FUNCTION "Gest Output" : VOID
TITLE =GESTIONE OUTPUT
AUTHOR : MassimoZ
VERSION : 0.1

BEGIN
NETWORK
TITLE =Spia Manuale
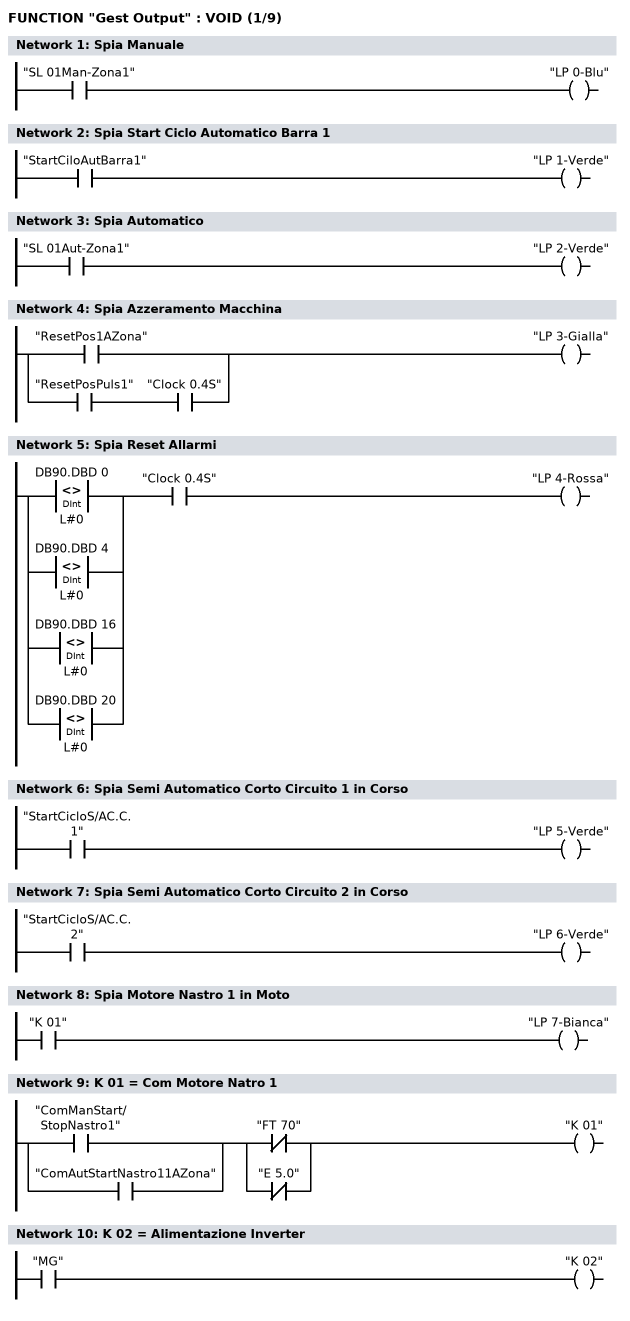
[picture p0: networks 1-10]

      U     "SL 01Man-Zona1";
      =     "LP 0-Blu";
NETWORK
TITLE =Spia Start Ciclo Automatico Barra 1

      U     "StartCiloAutBarra1";
      =     "LP 1-Verde";
NETWORK
TITLE =Spia Automatico

      U     "SL 01Aut-Zona1";
      =     "LP 2-Verde";
NETWORK
TITLE =Spia Azzeramento Macchina

      O     "ResetPos1AZona";
      O     ;
      U     "ResetPosPuls1";
      U     "Clock 0.4S";
      =     "LP 3-Gialla";
NETWORK
TITLE =Spia Reset Allarmi

      U(    ;
      O(    ;
      L     DB90.DBD    0;
      L     L#0;
      <>D   ;
      )     ;
      O(    ;
      L     DB90.DBD    4;
      L     L#0;
      <>D   ;
      )     ;
      O(    ;
      L     DB90.DBD   16;
      L     L#0;
      <>D   ;
      )     ;
      O(    ;
      L     DB90.DBD   20;
      L     L#0;
      <>D   ;
      )     ;
      )     ;
      U     "Clock 0.4S";
      =     "LP 4-Rossa";
NETWORK
TITLE =Spia Semi Automatico Corto Circuito 1 in Corso

      U     "StartCicloS/AC.C.1";
      =     "LP 5-Verde";
NETWORK
TITLE =Spia Semi Automatico Corto Circuito 2 in Corso

      U     "StartCicloS/AC.C.2";
      =     "LP 6-Verde";
NETWORK
TITLE =Spia Motore Nastro 1 in Moto

      U     "K 01";
      =     "LP 7-Bianca";
NETWORK
TITLE =K 01 = Com Motore Natro 1

      U(    ;
      O     "ComManStart/StopNastro1";
      O     "ComAutStartNastro11AZona";
      )     ;
      U(    ;
      ON    "FT 70";
      ON    "E       5.0";
      )     ;
      =     "K 01";
NETWORK
TITLE =K 02 = Alimentazione Inverter

      U     "MG";
      =     "K 02";
NETWORK
TITLE =K 03 = Com Motore Natro 3
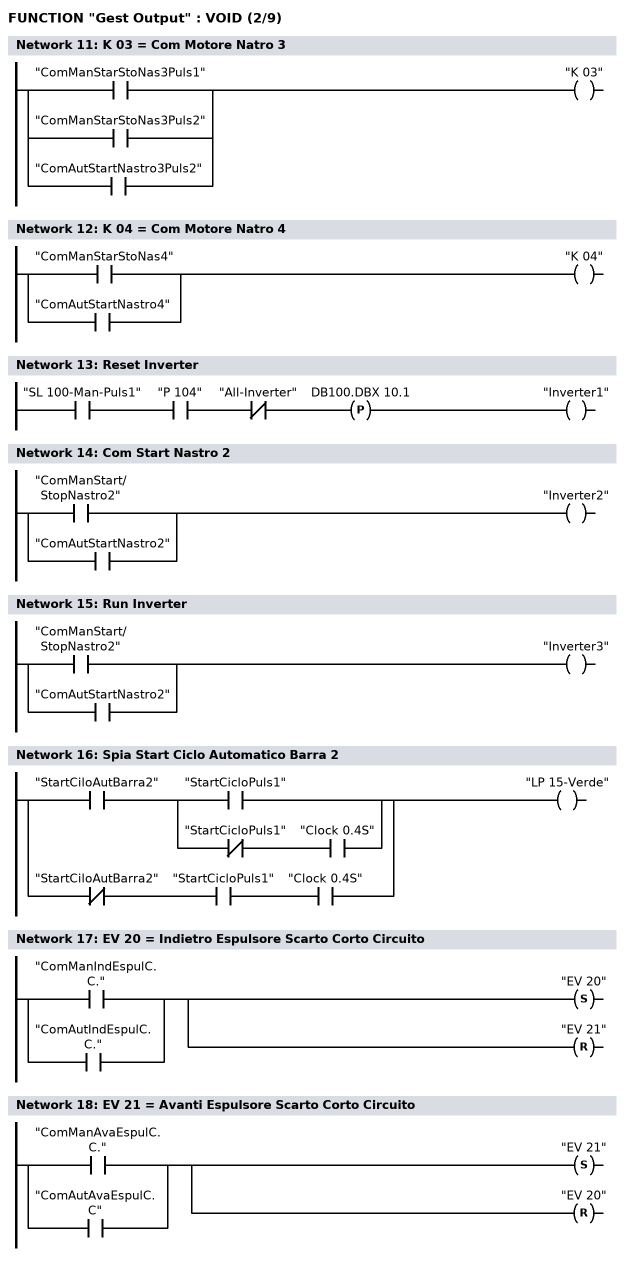
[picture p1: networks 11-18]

      O     "ComManStarStoNas3Puls1";
      O     "ComManStarStoNas3Puls2";
      O     "ComAutStartNastro3Puls2";
      =     "K 03";
NETWORK
TITLE =K 04 = Com Motore Natro 4

      O     "ComManStarStoNas4";
      O     "ComAutStartNastro4";
      =     "K 04";
NETWORK
TITLE =Reset Inverter

      U     "SL 100-Man-Puls1";
      U     "P 104";
      UN    "All-Inverter";
      FP    DB100.DBX   10.1;
      =     "Inverter1";
NETWORK
TITLE =Com Start Nastro 2

      O     "ComManStart/StopNastro2";
      O     "ComAutStartNastro2";
      =     "Inverter2";
NETWORK
TITLE =Run Inverter

      O     "ComManStart/StopNastro2";
      O     "ComAutStartNastro2";
      =     "Inverter3";
NETWORK
TITLE =Spia Start Ciclo Automatico Barra 2

      U     "StartCiloAutBarra2";
      U(    ;
      O     "StartCicloPuls1";
      O     ;
      UN    "StartCicloPuls1";
      U     "Clock 0.4S";
      )     ;
      O     ;
      UN    "StartCiloAutBarra2";
      U     "StartCicloPuls1";
      U     "Clock 0.4S";
      =     "LP 15-Verde";
NETWORK
TITLE =EV 20 = Indietro Espulsore Scarto Corto Circuito

      O     "ComManIndEspulC.C.";
      O     "ComAutIndEspulC.C.";
      S     "EV 20";
      R     "EV 21";
NETWORK
TITLE =EV 21 = Avanti Espulsore Scarto Corto Circuito

      O     "ComManAvaEspulC.C.";
      O     "ComAutAvaEspulC.C";
      S     "EV 21";
      R     "EV 20";
NETWORK
TITLE =EV 22 = Apertura Tampone Parzializzatore su Nastro 3
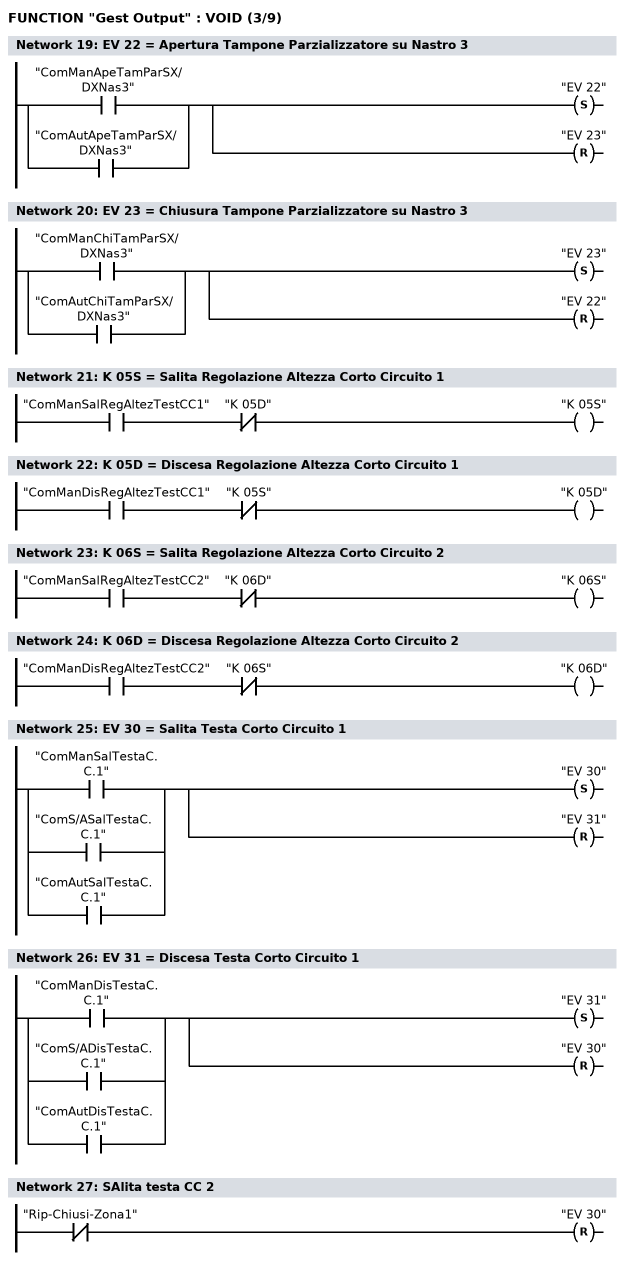
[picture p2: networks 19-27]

      O     "ComManApeTamParSX/DXNas3";
      O     "ComAutApeTamParSX/DXNas3";
      S     "EV 22";
      R     "EV 23";
NETWORK
TITLE =EV 23 = Chiusura Tampone Parzializzatore su Nastro 3

      O     "ComManChiTamParSX/DXNas3";
      O     "ComAutChiTamParSX/DXNas3";
      S     "EV 23";
      R     "EV 22";
NETWORK
TITLE =K 05S = Salita Regolazione Altezza Corto Circuito 1

      U     "ComManSalRegAltezTestCC1";
      UN    "K 05D";
      =     "K 05S";
NETWORK
TITLE =K 05D = Discesa Regolazione Altezza Corto Circuito 1

      U     "ComManDisRegAltezTestCC1";
      UN    "K 05S";
      =     "K 05D";
NETWORK
TITLE =K 06S = Salita Regolazione Altezza Corto Circuito 2

      U     "ComManSalRegAltezTestCC2";
      UN    "K 06D";
      =     "K 06S";
NETWORK
TITLE =K 06D = Discesa Regolazione Altezza Corto Circuito 2

      U     "ComManDisRegAltezTestCC2";
      UN    "K 06S";
      =     "K 06D";
NETWORK
TITLE =EV 30 = Salita Testa Corto Circuito 1

      O     "ComManSalTestaC.C.1";
      O     "ComS/ASalTestaC.C.1";
      O     "ComAutSalTestaC.C.1";
      S     "EV 30";
      R     "EV 31";
NETWORK
TITLE =EV 31 = Discesa Testa Corto Circuito 1

      O     "ComManDisTestaC.C.1";
      O     "ComS/ADisTestaC.C.1";
      O     "ComAutDisTestaC.C.1";
      S     "EV 31";
      R     "EV 30";
NETWORK
TITLE =SAlita testa CC 2

      UN    "Rip-Chiusi-Zona1";
      R     "EV 30";
NETWORK
TITLE =EV 32 = Salita Testa Corto Circuito 2
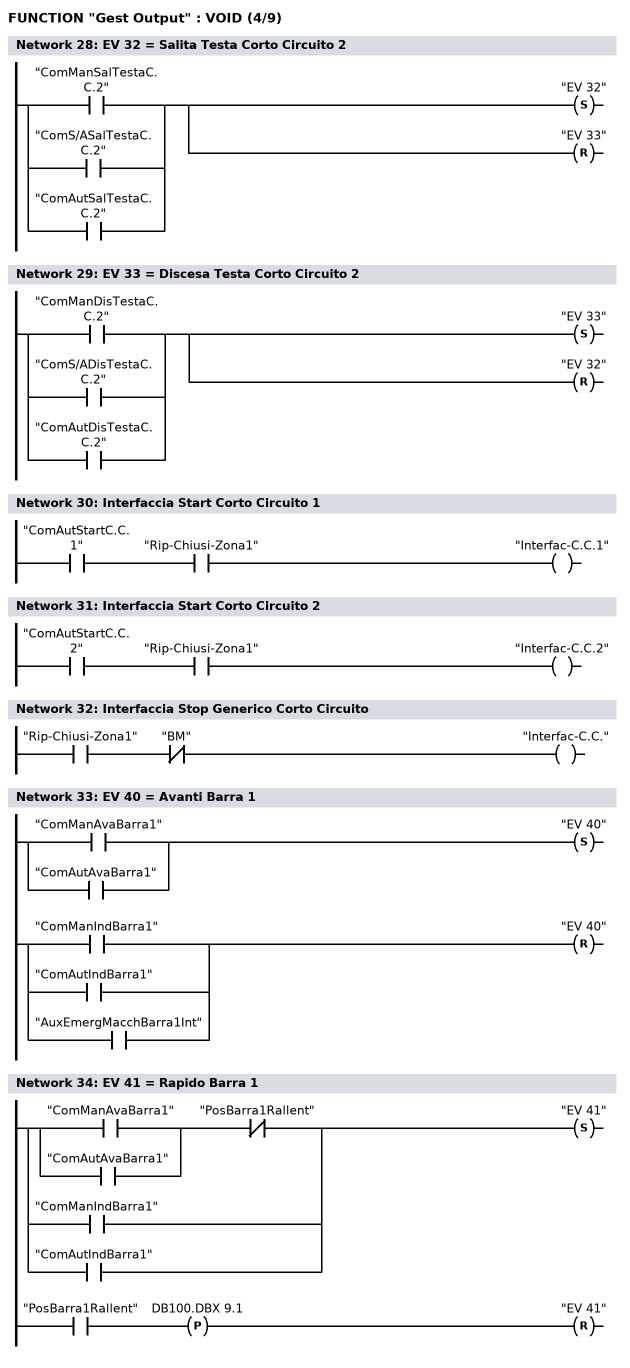
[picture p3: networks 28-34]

      O     "ComManSalTestaC.C.2";
      O     "ComS/ASalTestaC.C.2";
      O     "ComAutSalTestaC.C.2";
      S     "EV 32";
      R     "EV 33";
NETWORK
TITLE =EV 33 = Discesa Testa Corto Circuito 2

      O     "ComManDisTestaC.C.2";
      O     "ComS/ADisTestaC.C.2";
      O     "ComAutDisTestaC.C.2";
      S     "EV 33";
      R     "EV 32";
NETWORK
TITLE =Interfaccia Start Corto Circuito 1

      U     "ComAutStartC.C.1";
      U     "Rip-Chiusi-Zona1";
      =     "Interfac-C.C.1";
NETWORK
TITLE =Interfaccia Start Corto Circuito 2

      U     "ComAutStartC.C.2";
      U     "Rip-Chiusi-Zona1";
      =     "Interfac-C.C.2";
NETWORK
TITLE =Interfaccia Stop Generico Corto Circuito

      U     "Rip-Chiusi-Zona1";
      UN    "BM";
      =     "Interfac-C.C.";
NETWORK
TITLE =EV 40 = Avanti Barra 1

      U(    ;
      O     "ComManAvaBarra1";
      O     "ComAutAvaBarra1";
      )     ;
      S     "EV 40";
      U(    ;
      O     "ComManIndBarra1";
      O     "ComAutIndBarra1";
      O     "AuxEmergMacchBarra1Int";
      )     ;
      R     "EV 40";
      NOP   0;
NETWORK
TITLE =EV 41 = Rapido Barra 1

      U(    ;
      U(    ;
      O     "ComManAvaBarra1";
      O     "ComAutAvaBarra1";
      )     ;
      UN    "PosBarra1Rallent";
      O     "ComManIndBarra1";
      O     "ComAutIndBarra1";
      )     ;
      S     "EV 41";
      U     "PosBarra1Rallent";
      FP    DB100.DBX    9.1;
      R     "EV 41";
      NOP   0;
NETWORK
TITLE =EV 42 = Avanti Barra 2
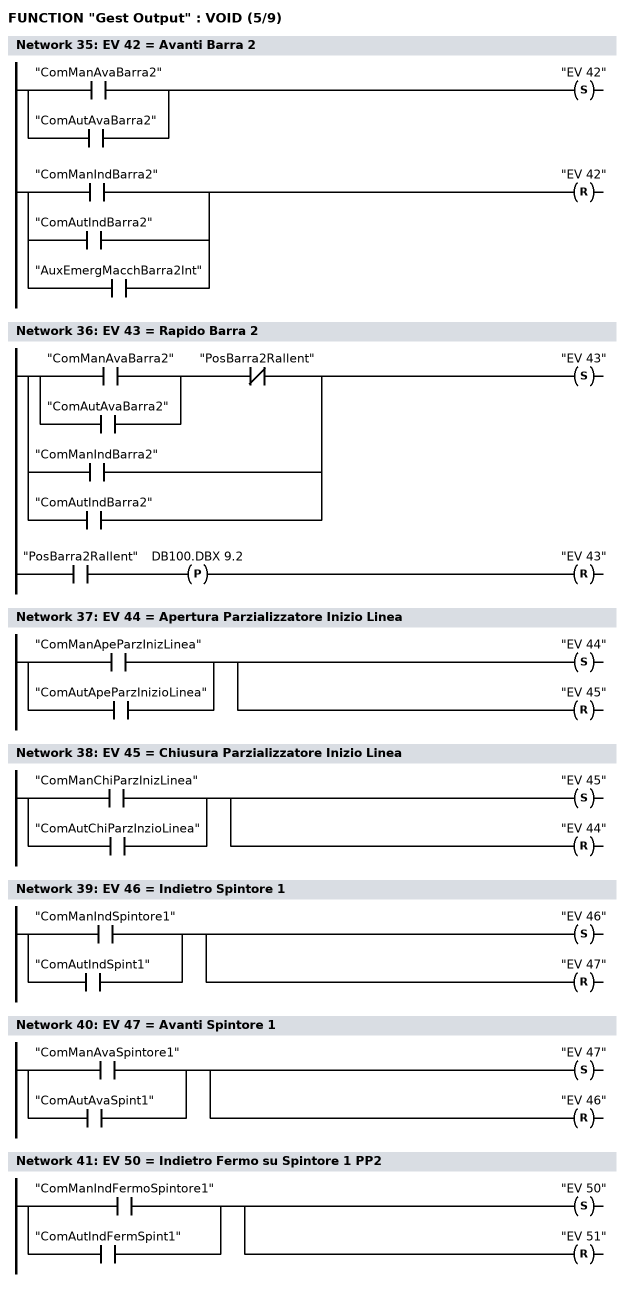
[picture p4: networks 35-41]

      U(    ;
      O     "ComManAvaBarra2";
      O     "ComAutAvaBarra2";
      )     ;
      S     "EV 42";
      U(    ;
      O     "ComManIndBarra2";
      O     "ComAutIndBarra2";
      O     "AuxEmergMacchBarra2Int";
      )     ;
      R     "EV 42";
      NOP   0;
NETWORK
TITLE =EV 43 = Rapido Barra 2

      U(    ;
      U(    ;
      O     "ComManAvaBarra2";
      O     "ComAutAvaBarra2";
      )     ;
      UN    "PosBarra2Rallent";
      O     "ComManIndBarra2";
      O     "ComAutIndBarra2";
      )     ;
      S     "EV 43";
      U     "PosBarra2Rallent";
      FP    DB100.DBX    9.2;
      R     "EV 43";
      NOP   0;
NETWORK
TITLE =EV 44 = Apertura Parzializzatore Inizio Linea

      O     "ComManApeParzInizLinea";
      O     "ComAutApeParzInizioLinea";
      S     "EV 44";
      R     "EV 45";
NETWORK
TITLE =EV 45 = Chiusura Parzializzatore Inizio Linea

      O     "ComManChiParzInizLinea";
      O     "ComAutChiParzInzioLinea";
      S     "EV 45";
      R     "EV 44";
NETWORK
TITLE =EV 46 = Indietro Spintore 1

      O     "ComManIndSpintore1";
      O     "ComAutIndSpint1";
      S     "EV 46";
      R     "EV 47";
NETWORK
TITLE =EV 47 = Avanti Spintore 1

      O     "ComManAvaSpintore1";
      O     "ComAutAvaSpint1";
      S     "EV 47";
      R     "EV 46";
NETWORK
TITLE =EV 50 = Indietro Fermo su Spintore 1 PP2

      O     "ComManIndFermoSpintore1";
      O     "ComAutIndFermSpint1";
      S     "EV 50";
      R     "EV 51";
NETWORK
TITLE =EV 51 = Avanti Fermo su Spintore 1 PP2
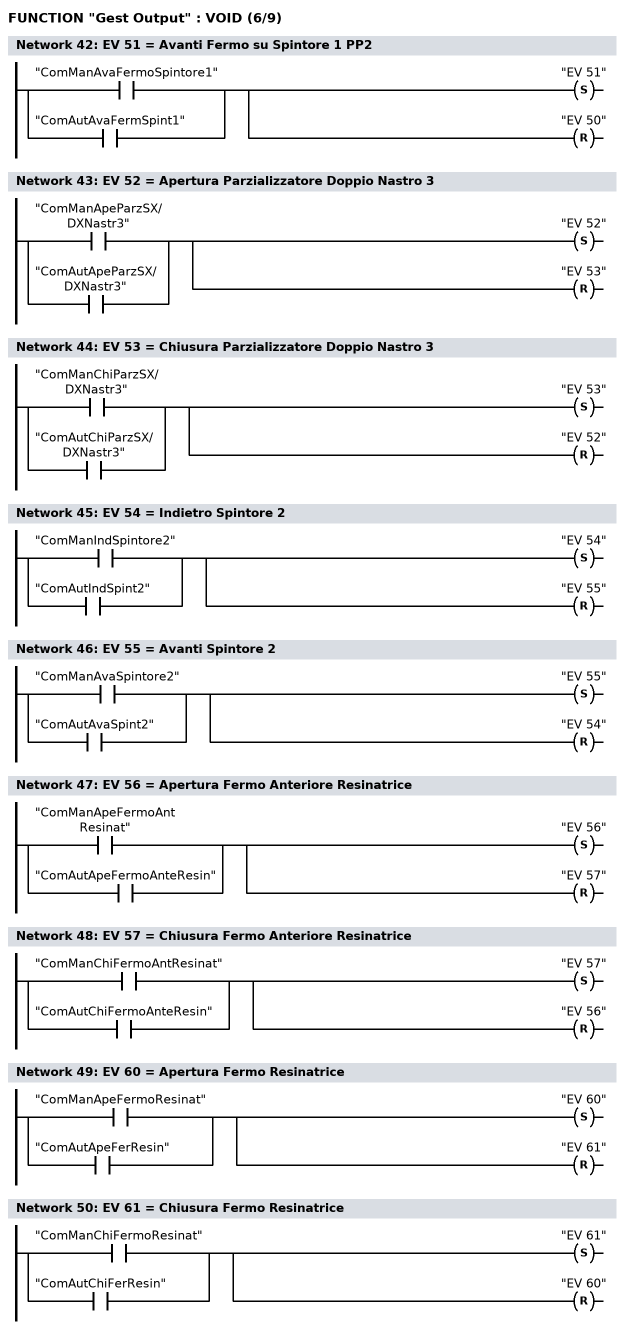
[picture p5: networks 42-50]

      O     "ComManAvaFermoSpintore1";
      O     "ComAutAvaFermSpint1";
      S     "EV 51";
      R     "EV 50";
NETWORK
TITLE =EV 52 = Apertura Parzializzatore Doppio Nastro 3

      O     "ComManApeParzSX/DXNastr3";
      O     "ComAutApeParzSX/DXNastr3";
      S     "EV 52";
      R     "EV 53";
NETWORK
TITLE =EV 53 = Chiusura Parzializzatore Doppio Nastro 3

      O     "ComManChiParzSX/DXNastr3";
      O     "ComAutChiParzSX/DXNastr3";
      S     "EV 53";
      R     "EV 52";
NETWORK
TITLE =EV 54 = Indietro Spintore 2

      O     "ComManIndSpintore2";
      O     "ComAutIndSpint2";
      S     "EV 54";
      R     "EV 55";
NETWORK
TITLE =EV 55 = Avanti Spintore 2

      O     "ComManAvaSpintore2";
      O     "ComAutAvaSpint2";
      S     "EV 55";
      R     "EV 54";
NETWORK
TITLE =EV 56 = Apertura Fermo Anteriore Resinatrice

      O     "ComManApeFermoAntResinat";
      O     "ComAutApeFermoAnteResin";
      S     "EV 56";
      R     "EV 57";
NETWORK
TITLE =EV 57 = Chiusura Fermo Anteriore Resinatrice

      O     "ComManChiFermoAntResinat";
      O     "ComAutChiFermoAnteResin";
      S     "EV 57";
      R     "EV 56";
NETWORK
TITLE =EV 60 = Apertura Fermo Resinatrice

      O     "ComManApeFermoResinat";
      O     "ComAutApeFerResin";
      S     "EV 60";
      R     "EV 61";
NETWORK
TITLE =EV 61 = Chiusura Fermo Resinatrice

      O     "ComManChiFermoResinat";
      O     "ComAutChiFerResin";
      S     "EV 61";
      R     "EV 60";
NETWORK
TITLE =EV 62 = Apertura Bloccaggio Resinatrice
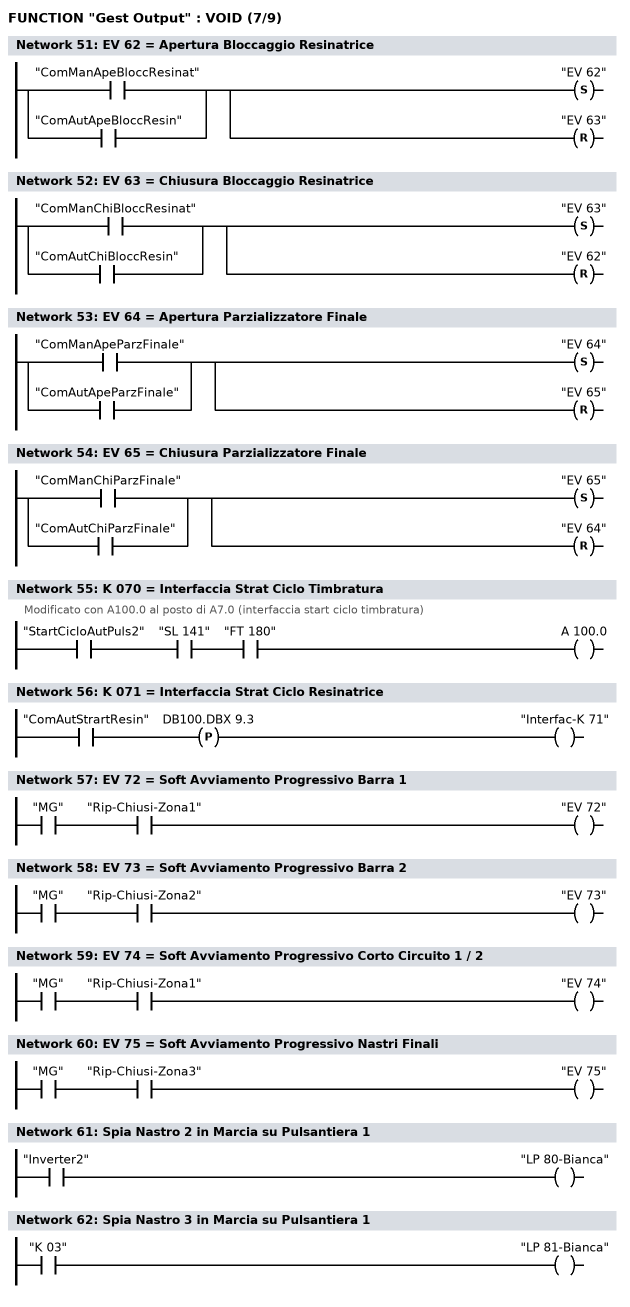
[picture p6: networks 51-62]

      O     "ComManApeBloccResinat";
      O     "ComAutApeBloccResin";
      S     "EV 62";
      R     "EV 63";
NETWORK
TITLE =EV 63 = Chiusura Bloccaggio Resinatrice

      O     "ComManChiBloccResinat";
      O     "ComAutChiBloccResin";
      S     "EV 63";
      R     "EV 62";
NETWORK
TITLE =EV 64 = Apertura Parzializzatore Finale

      O     "ComManApeParzFinale";
      O     "ComAutApeParzFinale";
      S     "EV 64";
      R     "EV 65";
NETWORK
TITLE =EV 65 = Chiusura Parzializzatore Finale

      O     "ComManChiParzFinale";
      O     "ComAutChiParzFinale";
      S     "EV 65";
      R     "EV 64";
NETWORK
TITLE =K 070 = Interfaccia Strat Ciclo Timbratura
//Modificato con A100.0 al posto di A7.0 (interfaccia start ciclo timbratura)
      U     "StartCicloAutPuls2";
      U     "SL 141";
      U     "FT 180";
      =     A    100.0;
NETWORK
TITLE =K 071 = Interfaccia Strat Ciclo Resinatrice

      U     "ComAutStrartResin";
      FP    DB100.DBX    9.3;
      =     "Interfac-K 71";
NETWORK
TITLE =EV 72 = Soft Avviamento Progressivo Barra 1

      U     "MG";
      U     "Rip-Chiusi-Zona1";
      =     "EV 72";
NETWORK
TITLE =EV 73 = Soft Avviamento Progressivo Barra 2

      U     "MG";
      U     "Rip-Chiusi-Zona2";
      =     "EV 73";
NETWORK
TITLE =EV 74 = Soft Avviamento Progressivo Corto Circuito 1 / 2

      U     "MG";
      U     "Rip-Chiusi-Zona1";
      =     "EV 74";
NETWORK
TITLE =EV 75 = Soft Avviamento Progressivo Nastri Finali

      U     "MG";
      U     "Rip-Chiusi-Zona3";
      =     "EV 75";
NETWORK
TITLE =Spia Nastro 2 in Marcia su Pulsantiera 1

      U     "Inverter2";
      =     "LP 80-Bianca";
NETWORK
TITLE =Spia Nastro 3 in Marcia su Pulsantiera 1

      U     "K 03";
      =     "LP 81-Bianca";
NETWORK
TITLE =Spia Reset Allarmi su Pulsantiera 1
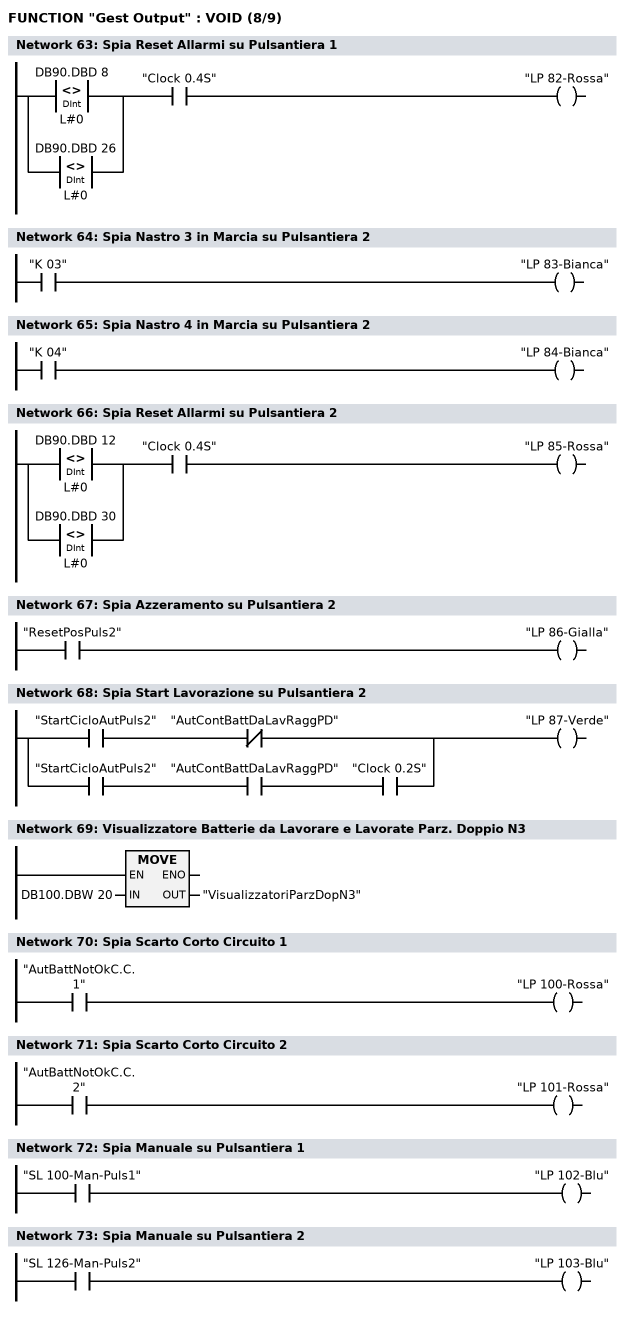
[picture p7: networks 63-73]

      U(    ;
      O(    ;
      L     DB90.DBD    8;
      L     L#0;
      <>D   ;
      )     ;
      O(    ;
      L     DB90.DBD   26;
      L     L#0;
      <>D   ;
      )     ;
      )     ;
      U     "Clock 0.4S";
      =     "LP 82-Rossa";
NETWORK
TITLE =Spia Nastro 3 in Marcia su Pulsantiera 2

      U     "K 03";
      =     "LP 83-Bianca";
NETWORK
TITLE =Spia Nastro 4 in Marcia su Pulsantiera 2

      U     "K 04";
      =     "LP 84-Bianca";
NETWORK
TITLE =Spia Reset Allarmi su Pulsantiera 2

      U(    ;
      O(    ;
      L     DB90.DBD   12;
      L     L#0;
      <>D   ;
      )     ;
      O(    ;
      L     DB90.DBD   30;
      L     L#0;
      <>D   ;
      )     ;
      )     ;
      U     "Clock 0.4S";
      =     "LP 85-Rossa";
NETWORK
TITLE =Spia Azzeramento su Pulsantiera 2

      U     "ResetPosPuls2";
      =     "LP 86-Gialla";
NETWORK
TITLE =Spia Start Lavorazione su Pulsantiera 2

      U     "StartCicloAutPuls2";
      UN    "AutContBattDaLavRaggPD";
      O     ;
      U     "StartCicloAutPuls2";
      U     "AutContBattDaLavRaggPD";
      U     "Clock 0.2S";
      =     "LP 87-Verde";
NETWORK
TITLE =Visualizzatore Batterie da Lavorare e Lavorate Parz. Doppio N3


      L     DB100.DBW   20;
      T     "VisualizzatoriParzDopN3";
      NOP   0;
NETWORK
TITLE =Spia Scarto Corto Circuito 1

      U     "AutBattNotOkC.C.1";
      =     "LP 100-Rossa";
NETWORK
TITLE =Spia Scarto Corto Circuito 2

      U     "AutBattNotOkC.C.2";
      =     "LP 101-Rossa";
NETWORK
TITLE =Spia Manuale su Pulsantiera 1

      U     "SL 100-Man-Puls1";
      =     "LP 102-Blu";
NETWORK
TITLE =Spia Manuale su Pulsantiera 2

      U     "SL 126-Man-Puls2";
      =     "LP 103-Blu";
NETWORK
TITLE =Spia Automatico su Pulsantiera 1
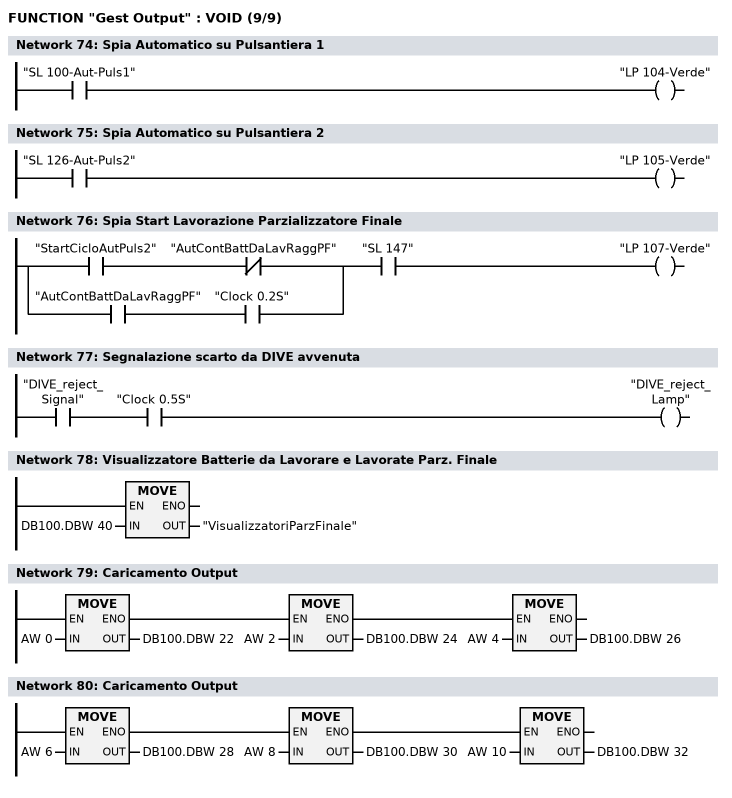
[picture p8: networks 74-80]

      U     "SL 100-Aut-Puls1";
      =     "LP 104-Verde";
NETWORK
TITLE =Spia Automatico su Pulsantiera 2

      U     "SL 126-Aut-Puls2";
      =     "LP 105-Verde";
NETWORK
TITLE =Spia Start Lavorazione Parzializzatore Finale

      U(    ;
      U     "StartCicloAutPuls2";
      UN    "AutContBattDaLavRaggPF";
      O     ;
      U     "AutContBattDaLavRaggPF";
      U     "Clock 0.2S";
      )     ;
      U     "SL 147";
      =     "LP 107-Verde";
NETWORK
TITLE =Segnalazione scarto da DIVE avvenuta

      U     "DIVE_reject_Signal";
      U     "Clock 0.5S";
      =     "DIVE_reject_Lamp";
NETWORK
TITLE =Visualizzatore Batterie da Lavorare e Lavorate Parz. Finale

      L     DB100.DBW   40;
      T     "VisualizzatoriParzFinale";
      NOP   0;
NETWORK
TITLE =Caricamento Output

      U(    ;
      U(    ;
      L     AW     0;
      T     DB100.DBW   22;
      SET   ;
      SAVE  ;
      CLR   ;
      U     BIE;
      )     ;
      SPBNB _001;
      L     AW     2;
      T     DB100.DBW   24;
      SET   ;
      SAVE  ;
      CLR   ;
_001: U     BIE;
      )     ;
      SPBNB _002;
      L     AW     4;
      T     DB100.DBW   26;
_002: NOP   0;
NETWORK
TITLE =Caricamento Output

      U(    ;
      U(    ;
      L     AW     6;
      T     DB100.DBW   28;
      SET   ;
      SAVE  ;
      CLR   ;
      U     BIE;
      )     ;
      SPBNB _003;
      L     AW     8;
      T     DB100.DBW   30;
      SET   ;
      SAVE  ;
      CLR   ;
_003: U     BIE;
      )     ;
      SPBNB _004;
      L     AW    10;
      T     DB100.DBW   32;
_004: NOP   0;
END_FUNCTION

